FUNCTION "Gest Avvisi Allarmi" : VOID
TITLE =Gestione Avvisi e Allarmi
AUTHOR : MassimoZ
FAMILY : NovaSrl
VERSION : 0.1

BEGIN
NETWORK
TITLE ======== Gestione Avvisi =======



NETWORK
TITLE =Avviso: Manca Marcia Generale
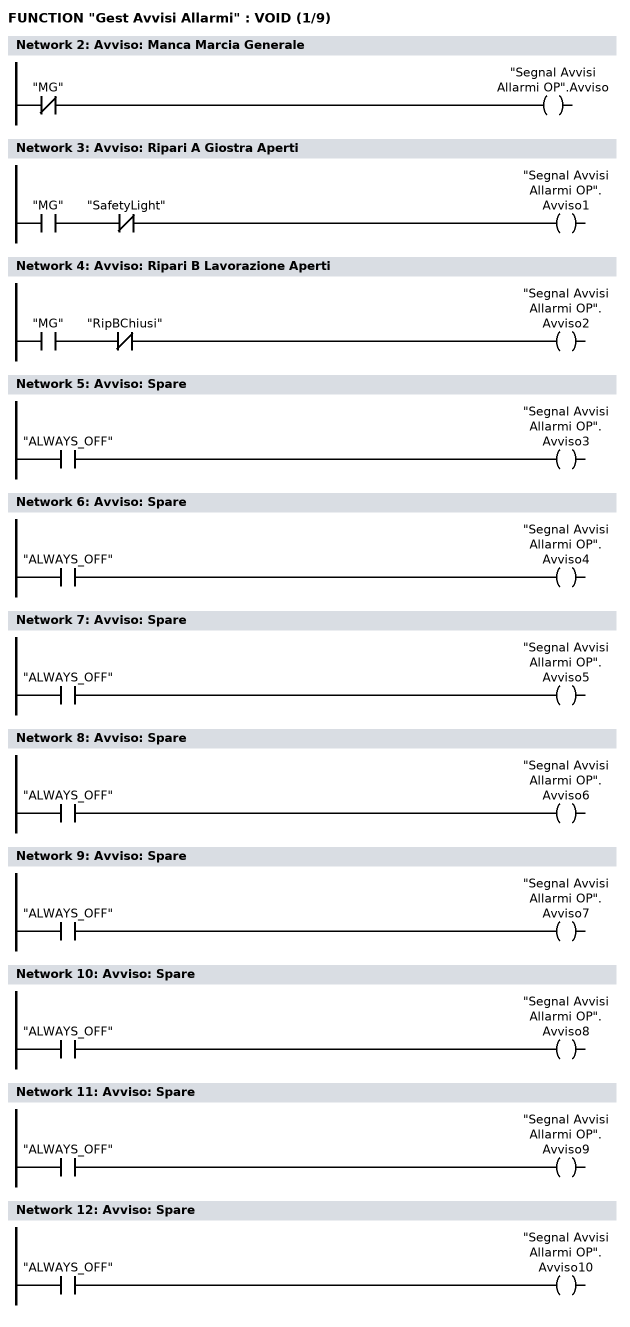
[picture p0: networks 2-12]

      UN    "MG";
      =     "Segnal Avvisi Allarmi OP".Avviso;
NETWORK
TITLE =Avviso: Ripari A Giostra Aperti

      U     "MG";
      UN    "SafetyLight";
      =     "Segnal Avvisi Allarmi OP".Avviso1;
NETWORK
TITLE =Avviso: Ripari B Lavorazione Aperti

      U     "MG";
      UN    "RipBChiusi";
      =     "Segnal Avvisi Allarmi OP".Avviso2;
NETWORK
TITLE =Avviso: Spare

      U     "ALWAYS_OFF";
      =     "Segnal Avvisi Allarmi OP".Avviso3;
NETWORK
TITLE =Avviso: Spare

      U     "ALWAYS_OFF";
      =     "Segnal Avvisi Allarmi OP".Avviso4;
NETWORK
TITLE =Avviso: Spare

      U     "ALWAYS_OFF";
      =     "Segnal Avvisi Allarmi OP".Avviso5;
NETWORK
TITLE =Avviso: Spare

      U     "ALWAYS_OFF";
      =     "Segnal Avvisi Allarmi OP".Avviso6;
NETWORK
TITLE =Avviso: Spare

      U     "ALWAYS_OFF";
      =     "Segnal Avvisi Allarmi OP".Avviso7;
NETWORK
TITLE =Avviso: Spare

      U     "ALWAYS_OFF";
      =     "Segnal Avvisi Allarmi OP".Avviso8;
NETWORK
TITLE =Avviso: Spare

      U     "ALWAYS_OFF";
      =     "Segnal Avvisi Allarmi OP".Avviso9;
NETWORK
TITLE =Avviso: Spare

      U     "ALWAYS_OFF";
      =     "Segnal Avvisi Allarmi OP".Avviso10;
NETWORK
TITLE =Avviso: Spare
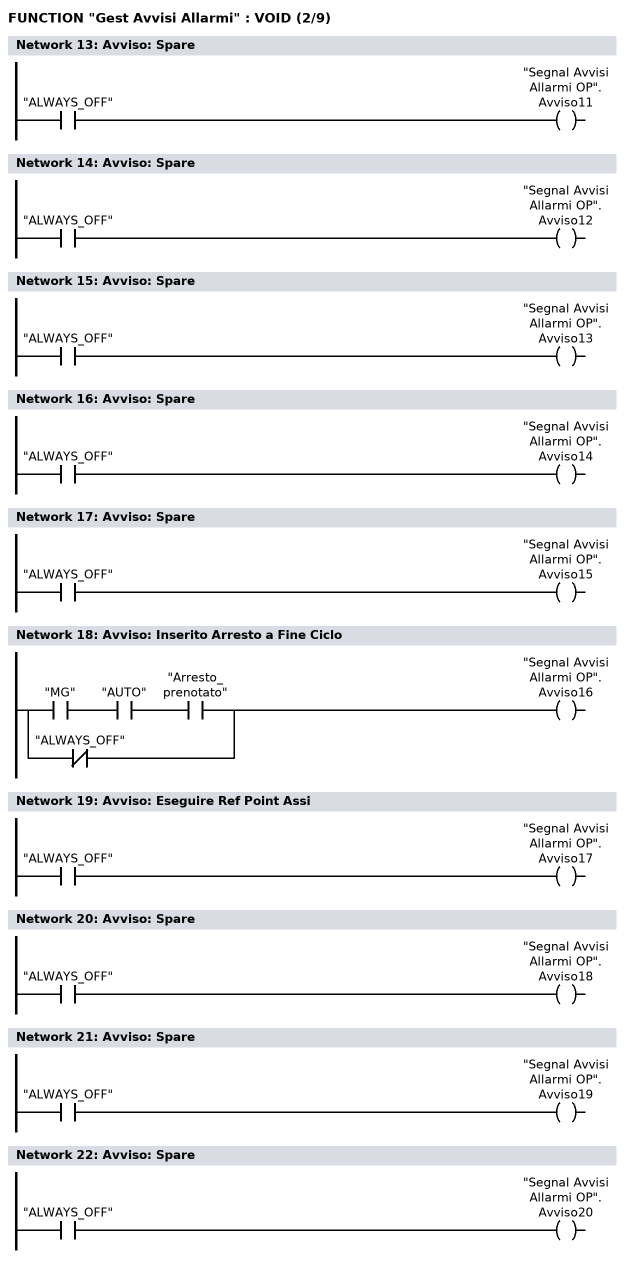
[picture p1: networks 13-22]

      U     "ALWAYS_OFF";
      =     "Segnal Avvisi Allarmi OP".Avviso11;
NETWORK
TITLE =Avviso: Spare

      U     "ALWAYS_OFF";
      =     "Segnal Avvisi Allarmi OP".Avviso12;
NETWORK
TITLE =Avviso: Spare

      U     "ALWAYS_OFF";
      =     "Segnal Avvisi Allarmi OP".Avviso13;
NETWORK
TITLE =Avviso: Spare

      U     "ALWAYS_OFF";
      =     "Segnal Avvisi Allarmi OP".Avviso14;
NETWORK
TITLE =Avviso: Spare

      U     "ALWAYS_OFF";
      =     "Segnal Avvisi Allarmi OP".Avviso15;
NETWORK
TITLE =Avviso: Inserito Arresto a Fine Ciclo

      U     "MG";
      U     "AUTO";
      U     "Arresto_prenotato";
      ON    "ALWAYS_OFF";
      =     "Segnal Avvisi Allarmi OP".Avviso16;
NETWORK
TITLE =Avviso: Eseguire Ref Point Assi

      U     "ALWAYS_OFF";
      =     "Segnal Avvisi Allarmi OP".Avviso17;
NETWORK
TITLE =Avviso: Spare

      U     "ALWAYS_OFF";
      =     "Segnal Avvisi Allarmi OP".Avviso18;
NETWORK
TITLE =Avviso: Spare

      U     "ALWAYS_OFF";
      =     "Segnal Avvisi Allarmi OP".Avviso19;
NETWORK
TITLE =Avviso: Spare

      U     "ALWAYS_OFF";
      =     "Segnal Avvisi Allarmi OP".Avviso20;
NETWORK
TITLE =Avviso: Spare
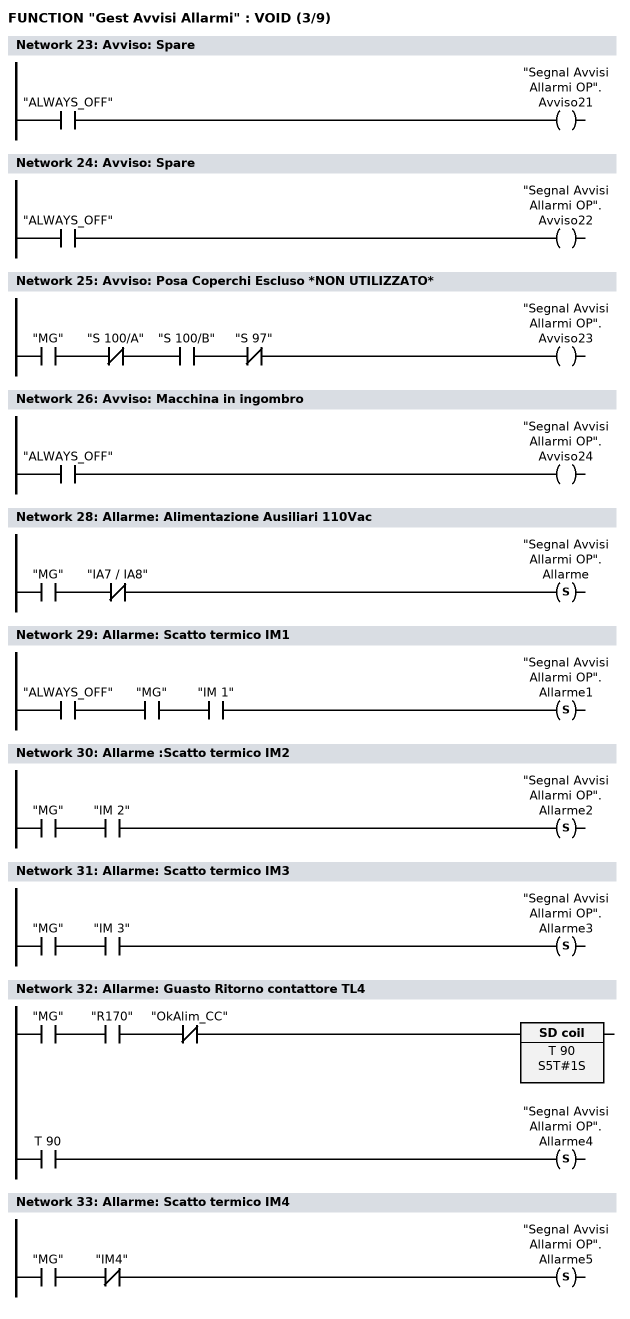
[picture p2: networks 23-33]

      U     "ALWAYS_OFF";
      =     "Segnal Avvisi Allarmi OP".Avviso21;
NETWORK
TITLE =Avviso: Spare

      U     "ALWAYS_OFF";
      =     "Segnal Avvisi Allarmi OP".Avviso22;
NETWORK
TITLE =Avviso: Posa Coperchi Escluso *NON UTILIZZATO*

      U     "MG";
      UN    "S 100/A";
      U     "S 100/B";
      UN    "S 97";
      =     "Segnal Avvisi Allarmi OP".Avviso23;
NETWORK
TITLE =Avviso: Macchina in ingombro

      U     "ALWAYS_OFF";
      =     "Segnal Avvisi Allarmi OP".Avviso24;
NETWORK
TITLE ======== Gestione Allarmi =======



NETWORK
TITLE =Allarme: Alimentazione Ausiliari 110Vac

      U     "MG";
      UN    "IA7 / IA8";
      S     "Segnal Avvisi Allarmi OP".Allarme;
NETWORK
TITLE =Allarme: Scatto termico IM1

      U     "ALWAYS_OFF";
      U     "MG";
      U     "IM 1";
      S     "Segnal Avvisi Allarmi OP".Allarme1;
NETWORK
TITLE =Allarme :Scatto termico IM2

      U     "MG";
      U     "IM 2";
      S     "Segnal Avvisi Allarmi OP".Allarme2;
NETWORK
TITLE =Allarme: Scatto termico IM3

      U     "MG";
      U     "IM 3";
      S     "Segnal Avvisi Allarmi OP".Allarme3;
NETWORK
TITLE =Allarme: Guasto Ritorno contattore TL4

      U     "MG";
      U     "R170";
      UN    "OkAlim_CC";
      L     S5T#1S;
      SE    T     90;
      NOP   0;
      NOP   0;
      NOP   0;
      U     T     90;
      S     "Segnal Avvisi Allarmi OP".Allarme4;
NETWORK
TITLE =Allarme: Scatto termico IM4

      U     "MG";
      UN    "IM4";
      S     "Segnal Avvisi Allarmi OP".Allarme5;
NETWORK
TITLE =Allarme: Spare
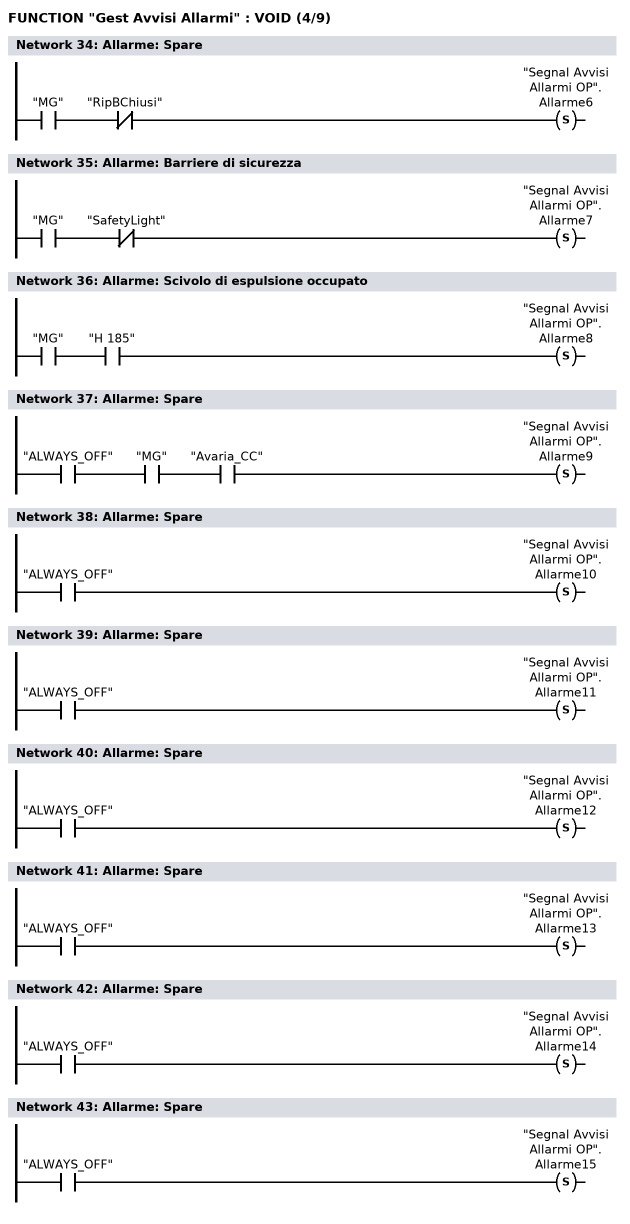
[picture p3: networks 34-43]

      U     "MG";
      UN    "RipBChiusi";
      S     "Segnal Avvisi Allarmi OP".Allarme6;
NETWORK
TITLE =Allarme: Barriere di sicurezza

      U     "MG";
      UN    "SafetyLight";
      S     "Segnal Avvisi Allarmi OP".Allarme7;
NETWORK
TITLE =Allarme: Scivolo di espulsione occupato

      U     "MG";
      U     "H 185";
      S     "Segnal Avvisi Allarmi OP".Allarme8;
NETWORK
TITLE =Allarme: Spare

      U     "ALWAYS_OFF";
      U     "MG";
      U     "Avaria_CC";
      S     "Segnal Avvisi Allarmi OP".Allarme9;
NETWORK
TITLE =Allarme: Spare

      U     "ALWAYS_OFF";
      S     "Segnal Avvisi Allarmi OP".Allarme10;
NETWORK
TITLE =Allarme: Spare

      U     "ALWAYS_OFF";
      S     "Segnal Avvisi Allarmi OP".Allarme11;
NETWORK
TITLE =Allarme: Spare

      U     "ALWAYS_OFF";
      S     "Segnal Avvisi Allarmi OP".Allarme12;
NETWORK
TITLE =Allarme: Spare

      U     "ALWAYS_OFF";
      S     "Segnal Avvisi Allarmi OP".Allarme13;
NETWORK
TITLE =Allarme: Spare

      U     "ALWAYS_OFF";
      S     "Segnal Avvisi Allarmi OP".Allarme14;
NETWORK
TITLE =Allarme: Spare

      U     "ALWAYS_OFF";
      S     "Segnal Avvisi Allarmi OP".Allarme15;
NETWORK
TITLE =Time Controllo Allarmi di Time-out
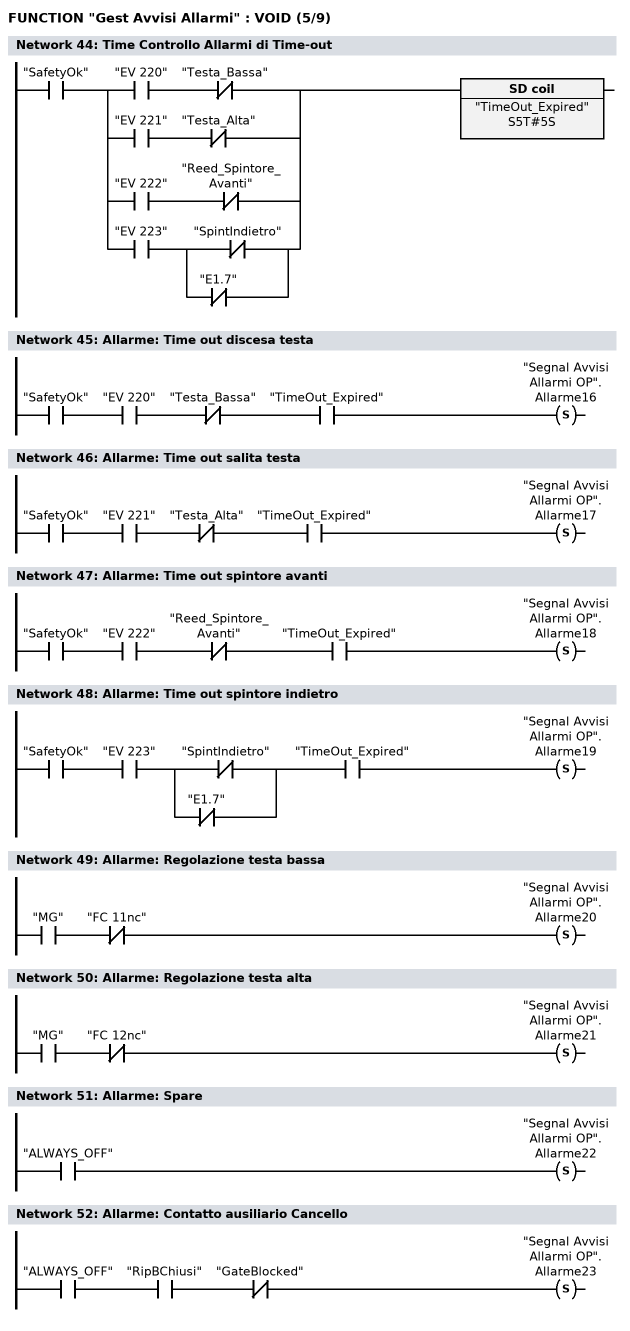
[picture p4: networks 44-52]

      U     "SafetyOk";
      U(    ;
      U     "EV 220";
      UN    "Testa_Bassa";
      O     ;
      U     "EV 221";
      UN    "Testa_Alta";
      O     ;
      U     "EV 222";
      UN    "Reed_Spintore_Avanti";
      O     ;
      U     "EV 223";
      U(    ;
      ON    "SpintIndietro";
      ON    "E1.7";
      )     ;
      )     ;
      L     S5T#5S;
      SE    "TimeOut_Expired";
      NOP   0;
      NOP   0;
      NOP   0;
      NOP   0;
NETWORK
TITLE =Allarme: Time out discesa testa

      U     "SafetyOk";
      U     "EV 220";
      UN    "Testa_Bassa";
      U     "TimeOut_Expired";
      S     "Segnal Avvisi Allarmi OP".Allarme16;
NETWORK
TITLE =Allarme: Time out salita testa

      U     "SafetyOk";
      U     "EV 221";
      UN    "Testa_Alta";
      U     "TimeOut_Expired";
      S     "Segnal Avvisi Allarmi OP".Allarme17;
NETWORK
TITLE =Allarme: Time out spintore avanti

      U     "SafetyOk";
      U     "EV 222";
      UN    "Reed_Spintore_Avanti";
      U     "TimeOut_Expired";
      S     "Segnal Avvisi Allarmi OP".Allarme18;
NETWORK
TITLE =Allarme: Time out spintore indietro

      U     "SafetyOk";
      U     "EV 223";
      U(    ;
      ON    "SpintIndietro";
      ON    "E1.7";
      )     ;
      U     "TimeOut_Expired";
      S     "Segnal Avvisi Allarmi OP".Allarme19;
NETWORK
TITLE =Allarme: Regolazione testa bassa

      U     "MG";
      UN    "FC 11nc";
      S     "Segnal Avvisi Allarmi OP".Allarme20;
NETWORK
TITLE =Allarme: Regolazione testa alta

      U     "MG";
      UN    "FC 12nc";
      S     "Segnal Avvisi Allarmi OP".Allarme21;
NETWORK
TITLE =Allarme: Spare

      U     "ALWAYS_OFF";
      S     "Segnal Avvisi Allarmi OP".Allarme22;
NETWORK
TITLE =Allarme: Contatto ausiliario Cancello

      U     "ALWAYS_OFF";
      U     "RipBChiusi";
      UN    "GateBlocked";
      S     "Segnal Avvisi Allarmi OP".Allarme23;
NETWORK
TITLE =Allarme: prenotazione arresto ciclo attivato
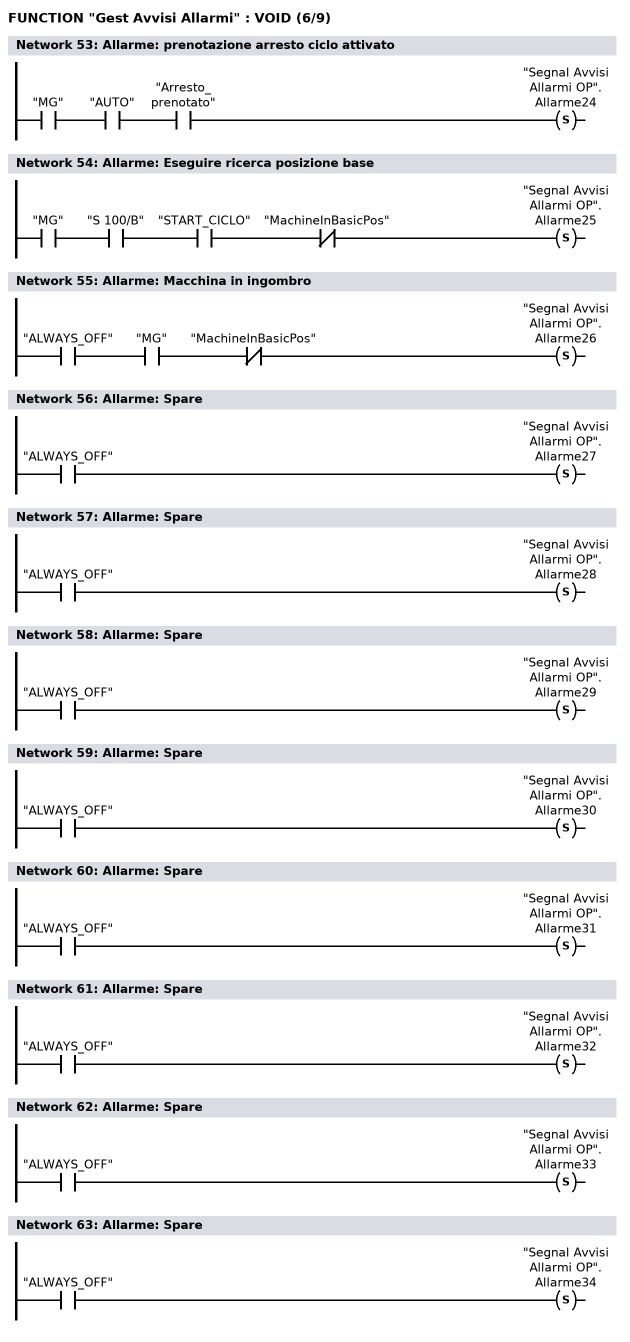
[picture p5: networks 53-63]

      U     "MG";
      U     "AUTO";
      U     "Arresto_prenotato";
      S     "Segnal Avvisi Allarmi OP".Allarme24;
NETWORK
TITLE =Allarme: Eseguire ricerca posizione base

      U     "MG";
      U     "S 100/B";
      U     "START_CICLO";
      UN    "MachineInBasicPos";
      S     "Segnal Avvisi Allarmi OP".Allarme25;
NETWORK
TITLE =Allarme: Macchina in ingombro

      U     "ALWAYS_OFF";
      U     "MG";
      UN    "MachineInBasicPos";
      S     "Segnal Avvisi Allarmi OP".Allarme26;
NETWORK
TITLE =Allarme: Spare

      U     "ALWAYS_OFF";
      S     "Segnal Avvisi Allarmi OP".Allarme27;
NETWORK
TITLE =Allarme: Spare

      U     "ALWAYS_OFF";
      S     "Segnal Avvisi Allarmi OP".Allarme28;
NETWORK
TITLE =Allarme: Spare

      U     "ALWAYS_OFF";
      S     "Segnal Avvisi Allarmi OP".Allarme29;
NETWORK
TITLE =Allarme: Spare

      U     "ALWAYS_OFF";
      S     "Segnal Avvisi Allarmi OP".Allarme30;
NETWORK
TITLE =Allarme: Spare

      U     "ALWAYS_OFF";
      S     "Segnal Avvisi Allarmi OP".Allarme31;
NETWORK
TITLE =Allarme: Spare

      U     "ALWAYS_OFF";
      S     "Segnal Avvisi Allarmi OP".Allarme32;
NETWORK
TITLE =Allarme: Spare

      U     "ALWAYS_OFF";
      S     "Segnal Avvisi Allarmi OP".Allarme33;
NETWORK
TITLE =Allarme: Spare

      U     "ALWAYS_OFF";
      S     "Segnal Avvisi Allarmi OP".Allarme34;
NETWORK
TITLE =Allarme: Spare
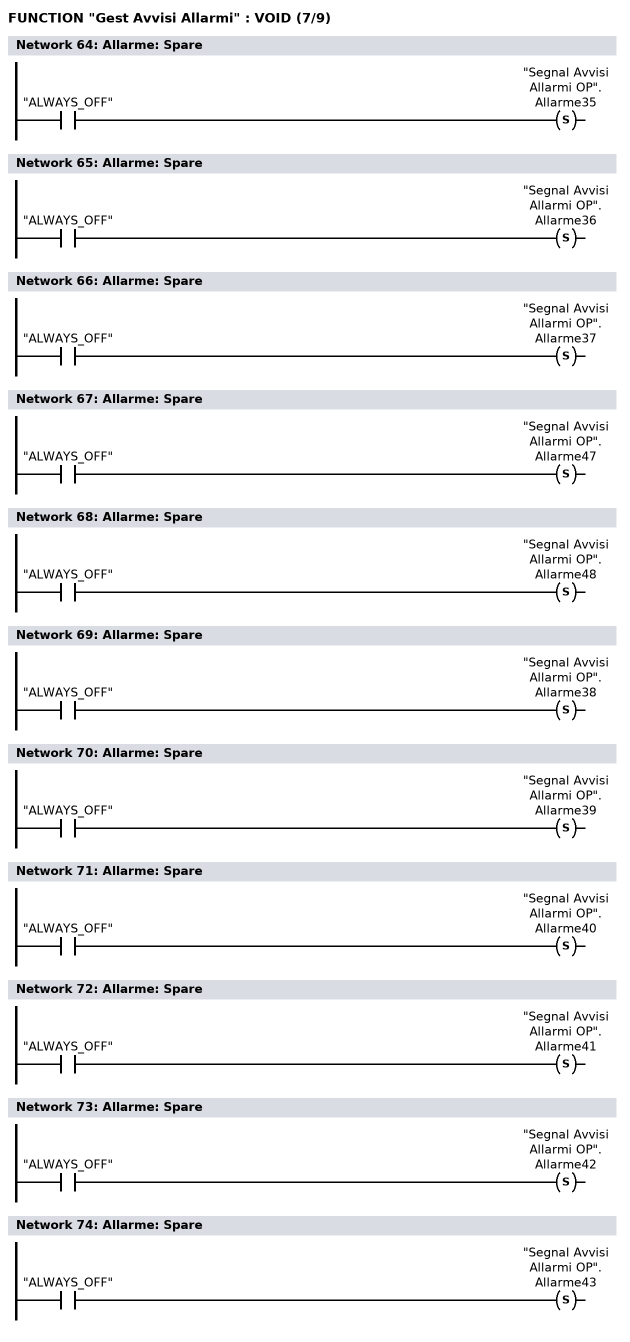
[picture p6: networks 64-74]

      U     "ALWAYS_OFF";
      S     "Segnal Avvisi Allarmi OP".Allarme35;
NETWORK
TITLE =Allarme: Spare

      U     "ALWAYS_OFF";
      S     "Segnal Avvisi Allarmi OP".Allarme36;
NETWORK
TITLE =Allarme: Spare

      U     "ALWAYS_OFF";
      S     "Segnal Avvisi Allarmi OP".Allarme37;
NETWORK
TITLE =Allarme: Spare

      U     "ALWAYS_OFF";
      S     "Segnal Avvisi Allarmi OP".Allarme47;
NETWORK
TITLE =Allarme: Spare

      U     "ALWAYS_OFF";
      S     "Segnal Avvisi Allarmi OP".Allarme48;
NETWORK
TITLE =Allarme: Spare

      U     "ALWAYS_OFF";
      S     "Segnal Avvisi Allarmi OP".Allarme38;
NETWORK
TITLE =Allarme: Spare

      U     "ALWAYS_OFF";
      S     "Segnal Avvisi Allarmi OP".Allarme39;
NETWORK
TITLE =Allarme: Spare

      U     "ALWAYS_OFF";
      S     "Segnal Avvisi Allarmi OP".Allarme40;
NETWORK
TITLE =Allarme: Spare

      U     "ALWAYS_OFF";
      S     "Segnal Avvisi Allarmi OP".Allarme41;
NETWORK
TITLE =Allarme: Spare

      U     "ALWAYS_OFF";
      S     "Segnal Avvisi Allarmi OP".Allarme42;
NETWORK
TITLE =Allarme: Spare

      U     "ALWAYS_OFF";
      S     "Segnal Avvisi Allarmi OP".Allarme43;
NETWORK
TITLE =Allarme: Spare
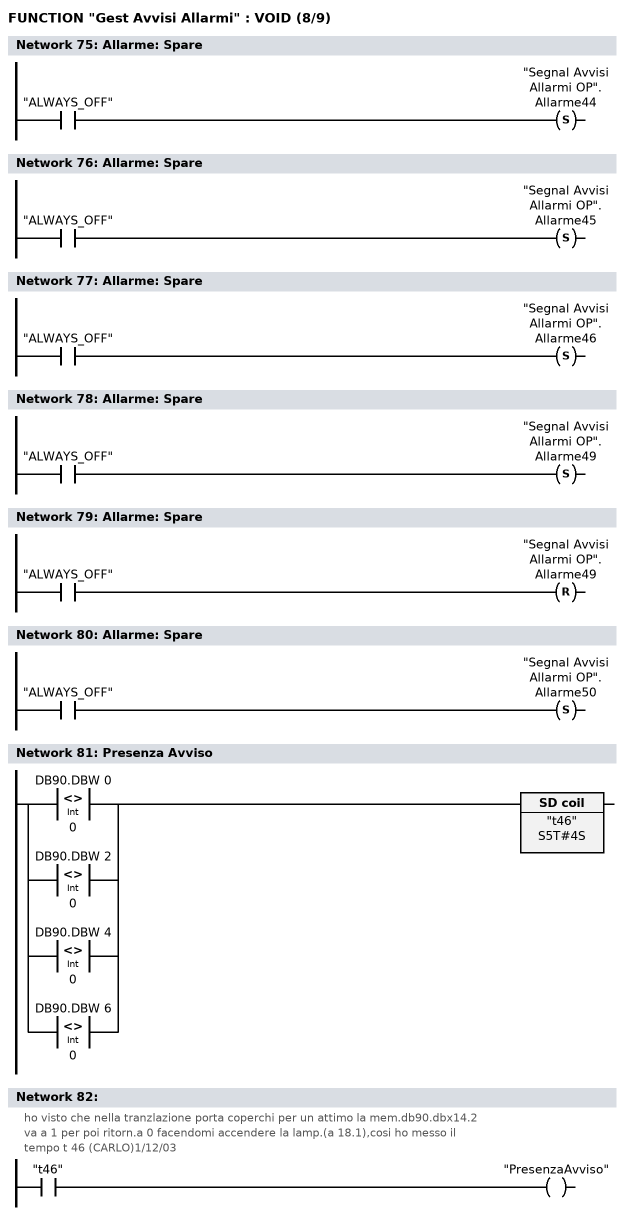
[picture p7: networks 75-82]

      U     "ALWAYS_OFF";
      S     "Segnal Avvisi Allarmi OP".Allarme44;
NETWORK
TITLE =Allarme: Spare

      U     "ALWAYS_OFF";
      S     "Segnal Avvisi Allarmi OP".Allarme45;
NETWORK
TITLE =Allarme: Spare

      U     "ALWAYS_OFF";
      S     "Segnal Avvisi Allarmi OP".Allarme46;
NETWORK
TITLE =Allarme: Spare

      U     "ALWAYS_OFF";
      S     "Segnal Avvisi Allarmi OP".Allarme49;
NETWORK
TITLE =Allarme: Spare

      U     "ALWAYS_OFF";
      R     "Segnal Avvisi Allarmi OP".Allarme49;
NETWORK
TITLE =Allarme: Spare

      U     "ALWAYS_OFF";
      S     "Segnal Avvisi Allarmi OP".Allarme50;

NETWORK
TITLE =Presenza Avviso

      O(    ;
      L     DB90.DBW    0;
      L     0;
      <>I   ;
      )     ;
      O(    ;
      L     DB90.DBW    2;
      L     0;
      <>I   ;
      )     ;
      O(    ;
      L     DB90.DBW    4;
      L     0;
      <>I   ;
      )     ;
      O(    ;
      L     DB90.DBW    6;
      L     0;
      <>I   ;
      )     ;
      L     S5T#4S;
      SE    "t46";

NETWORK
TITLE =
//ho visto che nella tranzlazione porta coperchi per un attimo la mem.db90.dbx14.2
//va a 1 per poi ritorn.a 0 facendomi accendere la lamp.(a 18.1),cosi ho messo il
//tempo t 46 (CARLO)1/12/03
      U     "t46";
      =     "PresenzaAvviso";

NETWORK
TITLE =Presenza Allarme
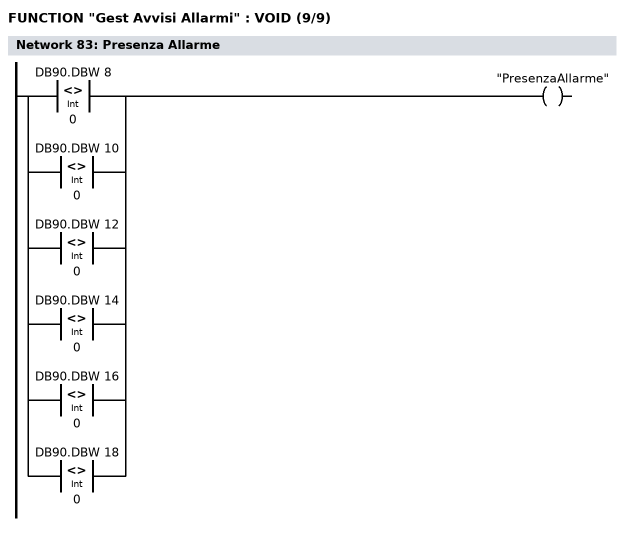
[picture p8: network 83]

      O(    ;
      L     DB90.DBW    8;
      L     0;
      <>I   ;
      )     ;
      O(    ;
      L     DB90.DBW   10;
      L     0;
      <>I   ;
      )     ;
      O(    ;
      L     DB90.DBW   12;
      L     0;
      <>I   ;
      )     ;
      O(    ;
      L     DB90.DBW   14;
      L     0;
      <>I   ;
      )     ;
      O(    ;
      L     DB90.DBW   16;
      L     0;
      <>I   ;
      )     ;
      O(    ;
      L     DB90.DBW   18;
      L     0;
      <>I   ;
      )     ;
      =     "PresenzaAllarme";
NETWORK
TITLE =Reset Allarmi

      U     "RESET_ALLARMI";
      FP    "FronteS/D-M251.6";
      SPBNB M001;
      L     0;
      T     DB90.DBW    8;
      T     DB90.DBW   10;
      T     DB90.DBW   12;
      T     DB90.DBW   14;
      T     DB90.DBW   16;
      T     DB90.DBW   18;
M001: NOP   0;

//ACQUISIZIONE ALLARMI DA PLC
      L     DB90.DBW    8;
      INVI  ;
      T     "Segnal Avvisi Allarmi OP".AcquPlc;

      L     DB90.DBW   10;
      INVI  ;
      T     "Segnal Avvisi Allarmi OP".AcquPlc1;

      L     DB90.DBW   12;
      INVI  ;
      T     "Segnal Avvisi Allarmi OP".AcquPlc2;

      L     DB90.DBW   14;
      INVI  ;
      T     "Segnal Avvisi Allarmi OP".AcquPlc3;

      L     DB90.DBW   16;
      INVI  ;
      T     "Segnal Avvisi Allarmi OP".AcquPlc4;

      L     DB90.DBW   18;
      INVI  ;
      T     "Segnal Avvisi Allarmi OP".AcquPlc5;
END_FUNCTION

